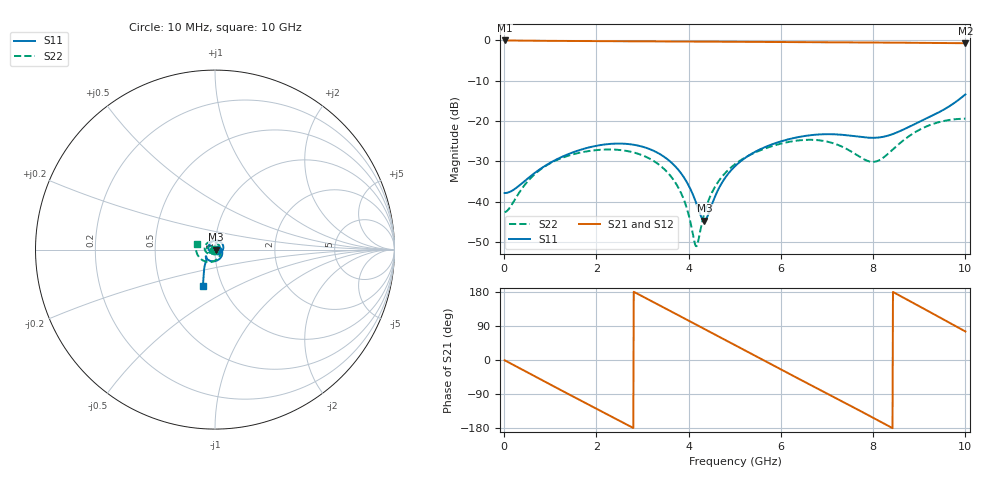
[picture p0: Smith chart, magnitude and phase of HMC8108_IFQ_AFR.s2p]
! Analog Devices, Inc.
! 1 Analog Way
! Wilmington, MA 01887
! http://www.analog.com
! Date:  2021-09-07 NN
! Board Name:  EV1HMC8108LC5 Revision A with HMC8108LC5 installed
! File Description:  Automatic Fixture Removal S-Parameters for IFQ Port connector and board loss de-embedding
! File Generation:  Calibrated Network Analyzer
! Chip Part Number:  HMC8108
! Chip Description:  X-Band, GaAs, MMIC, Low Noise Converter
! Chip Frequency:  9 to 10 GHz
! Chip Package:  LCC, 5 x 5 x 1.12 mm
! IFQ Port:  HMC8108LC5 removed and end of trace left open
! Note:
!  Analog Devices supplies this data as a sample of measured data at the evaluation board
!  ports for this product.  Your particular data for this product may vary.
!  Analog Devices reserves the right to change this data at anytime.
!  All lines below in this file are as is from the Network Analyzer.
!Agilent Technologies,N5245A,MY52451809,A.10.47.06
!Automatic Fixture Removal (AFR)
!Date: Friday, August 27, 2021 5:29:07 AM
!S2P File: Measurements: S11,S21,S12,S22:
# MHz S  RI  R 50
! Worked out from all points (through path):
!   1000 points, 10 MHz to 10 GHz, reference 50 ohm
!   highest |S21| = 0.00 dB at 10 MHz (marker M1); lowest = -0.7 dB at 10 GHz (marker M2)
!   group delay of S21, straight-line fit = 178 ps
!   lowest |S11| = -44.7 dB at 4.34 GHz (marker M3), VSWR 1.01, Z = 50.6 - j0.0657 ohm
!   |S11| at or under -10 dB: start of sweep to end of sweep
!   |S22| runs from -51.0 to -19.4 dB; largest |S21 - S12| = 1.4e-15
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10  0.0128 -0.000513  0.9999 -0.0113  0.9999 -0.0113  -0.00743 -0.000278
450  0.000169 -0.0182  0.8686 -0.4848  0.8686 -0.4848  -0.0116 -0.0114
930  -0.0259 -0.0128  0.4921 -0.8581  0.4921 -0.8581  -0.0225 -0.0175
1680  -0.0269 0.0355  -0.3076 -0.9346  -0.3076 -0.9346  -0.0395 -0.0113
2550  0.034 0.0402  -0.9374 -0.2775  -0.9374 -0.2775  -0.0422 0.0108
2940  0.0466 0.0158  -0.9647 0.1408  -0.9647 0.1408  -0.0336 0.0194
3340  0.0394 -0.00758  -0.8077 0.5416  -0.8077 0.5416  -0.0203 0.0212
3830  0.0169 -0.0153  -0.4049 0.881  -0.4049 0.881  -0.00615 0.0115
4150  0.00694 -0.00739  -0.0681 0.9653  -0.0681 0.9653  -0.00282 0.000513
4340  0.00581 -0.00065  0.1387 0.9566  0.1387 0.9566  -0.00363 -0.00623
4600  0.0104 0.00715  0.4089 0.8741  0.4089 0.8741  -0.00774 -0.0144
5010  0.0267 0.00771  0.7541 0.5984  0.7541 0.5984  -0.0191 -0.0224
5410  0.0396 -0.00934  0.9368 0.2109  0.9368 0.2109  -0.0326 -0.0234
5800  0.0373 -0.0353  0.9359 -0.2037  0.9359 -0.2037  -0.0455 -0.0176
6670  -0.0169 -0.065  0.3644 -0.8796  0.3644 -0.8796  -0.0548 0.0208
7050  -0.0396 -0.0564  -0.026 -0.9492  -0.026 -0.9492  -0.0381 0.0394
7440  -0.0506 -0.0434  -0.421 -0.8485  -0.421 -0.8485  -0.00792 0.044
7970  -0.0497 -0.0373  -0.8212 -0.4647  -0.8212 -0.4647  0.0288 0.0121
8340  -0.0476 -0.0465  -0.9364 -0.0886  -0.9364 -0.0886  0.029 -0.0278
8790  -0.0515 -0.0683  -0.854 0.384  -0.854 0.384  -0.00859 -0.0653
9270  -0.0593 -0.0997  -0.52 0.7722  -0.52 0.7722  -0.0695 -0.0589
10000  -0.0684 -0.2031  0.2351 0.8939  0.2351 0.8939  -0.1024 0.032
